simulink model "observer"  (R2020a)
settings: Solver=VariableStepAuto  StartTime=0.0  StopTime=10.0  RelTol=1e-3
PreLoadFcn:
  | initParams
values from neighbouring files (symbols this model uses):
  A = [-1 -2 1;0 -5 -1;0 0 -1]    [initParams.m]
  B = [1;2;1]    [initParams.m]
  C = [1 0]    [initParams.m]
  D = 0    [initParams.m]
  L = place(A',C',ev).'    [initParams.m]
  x0 = [0.2;0.1]    [initParams.m]
  x0s = [0;0]    [initParams.m]

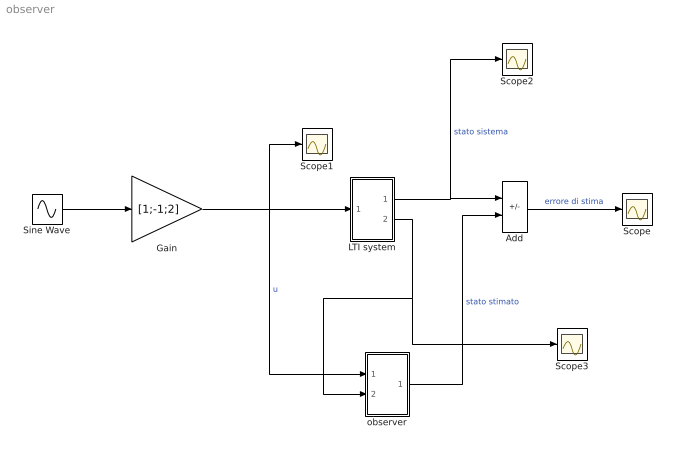
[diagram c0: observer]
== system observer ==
  Add : Sum  Inputs=+-
  Gain : Gain  Gain=[1;-1;2]  Multiplication=Matrix(K*u) (u vector)
  LTI system : Subsystem
  Scope{,1..3} (4 alike) : Scope
  Sine Wave : Sin  Phase=pi/2  SampleTime=0
  observer : Subsystem
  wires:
  LTI system/2(y) -> Scope3/1, observer/2(y)
  Gain/1 -> Scope1/1, observer/1(u), LTI system/1(u)  "u"
  LTI system/1(x) -> Scope2/1, Add/1  "stato sistema"
  observer/1(xHat) -> Add/2  "stato stimato"
  Add/1 -> Scope/1  "errore di stima"
  Sine Wave/1 -> Gain/1

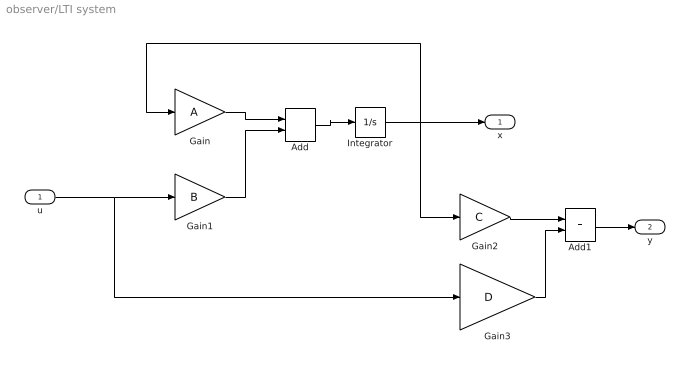
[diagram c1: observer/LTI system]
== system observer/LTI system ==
  u : Inport
  Add : Sum
  Add1 : Sum
  Gain : Gain  Gain=A  Multiplication=Matrix(K*u) (u vector)
  Gain1 : Gain  Gain=B  Multiplication=Matrix(K*u) (u vector)
  Gain2 : Gain  Gain=C  Multiplication=Matrix(K*u) (u vector)
  Gain3 : Gain  Gain=D  Multiplication=Matrix(K*u) (u vector)
  Integrator : Integrator  InitialCondition=x0
  x : Outport
  y : Outport  Port=2
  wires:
  Gain1/1 -> Add/2
  Integrator/1 -> x/1, Gain2/1, Gain/1
  Gain/1 -> Add/1
  Add/1 -> Integrator/1
  u/1 -> Gain3/1, Gain1/1
  Gain2/1 -> Add1/1
  Gain3/1 -> Add1/2
  Add1/1 -> y/1

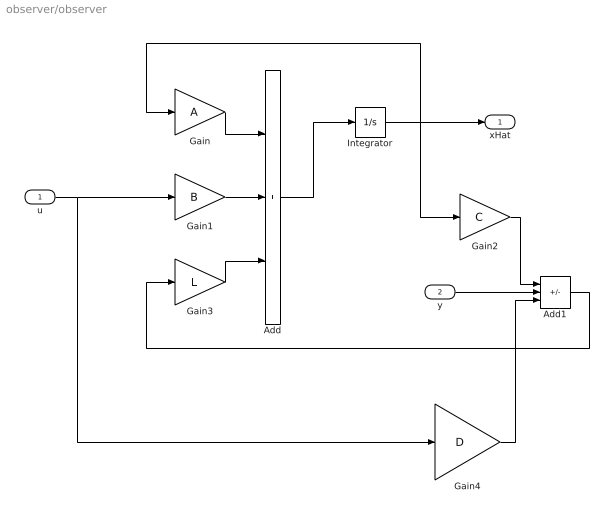
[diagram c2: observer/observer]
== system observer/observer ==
  u : Inport
  y : Inport  Port=2
  Add : Sum  Inputs=+++
  Add1 : Sum  Inputs=-+-
  Gain : Gain  Gain=A  Multiplication=Matrix(K*u) (u vector)
  Gain1 : Gain  Gain=B  Multiplication=Matrix(K*u) (u vector)
  Gain2 : Gain  Gain=C  Multiplication=Matrix(K*u) (u vector)
  Gain3 : Gain  Gain=L  Multiplication=Matrix(K*u) (u vector)
  Gain4 : Gain  Gain=D  Multiplication=Matrix(K*u) (u vector)
  Integrator : Integrator  InitialCondition=x0s
  xHat : Outport
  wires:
  Gain1/1 -> Add/2
  Integrator/1 -> xHat/1, Gain2/1, Gain/1
  Gain/1 -> Add/1
  Add/1 -> Integrator/1
  u/1 -> Gain4/1, Gain1/1
  Gain2/1 -> Add1/1
  y/1 -> Add1/2
  Gain3/1 -> Add/3
  Add1/1 -> Gain3/1
  Gain4/1 -> Add1/3
